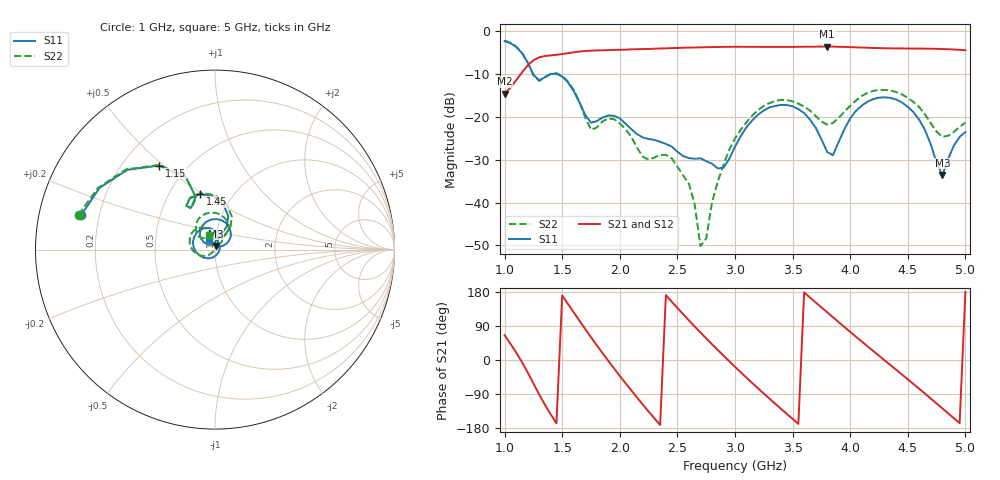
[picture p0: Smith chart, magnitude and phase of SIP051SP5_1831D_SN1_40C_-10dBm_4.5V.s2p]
# GHz  S  dB  R  50
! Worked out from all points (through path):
!   81 points, 1 GHz to 5 GHz, reference 50 ohm
!   highest |S21| = -3.53 dB at 3.8 GHz (marker M1); lowest = -14.5 dB at 1 GHz (marker M2)
!   lowest |S11| = -33.5 dB at 4.8 GHz (marker M3), VSWR 1.04, Z = 50.4 + j2.08 ohm
!   |S11| at or under -10 dB: 1.248 GHz to 1.397 GHz (148.8 MHz wide, 11.2 % of centre); 1.458 GHz to end of sweep
!   |S22| runs from -50.2 to -2.1 dB; largest |S21 - S12| = 0.0027
!   S11 on the Smith chart (normalised r, x): 1 GHz: 0.13, +0.13; 1.15 GHz: 0.35, +0.48; 1.45 GHz: 0.71, +0.49; 5 GHz: 0.93, +0.11
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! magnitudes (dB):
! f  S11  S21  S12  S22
! 1 GHz  -2.3  -14.5  -14.5  -2.1
! 1.15 GHz  -5.0  -9.6  -9.6  -5.0
! 1.3 GHz  -11.4  -6.0  -6.1  -11.6
! 1.45 GHz  -9.9  -5.5  -5.4  -9.7
! 1.7 GHz  -19.5  -4.6  -4.6  -20.1
! 1.75 GHz  -21.3  -4.5  -4.5  -22.9
! 1.95 GHz  -19.7  -4.3  -4.3  -20.5
! 2.2 GHz  -24.8  -4.1  -4.1  -29.3
! 2.35 GHz  -25.8  -4.0  -4.0  -28.9
! 2.6 GHz  -29.6  -3.8  -3.8  -35.6
! 2.7 GHz  -29.6  -3.7  -3.7  -50.2
! 2.75 GHz  -30.3  -3.7  -3.7  -48.4
! 2.9 GHz  -31.8  -3.6  -3.6  -31.2
! 3 GHz  -26.9  -3.6  -3.6  -25.0
! 3.35 GHz  -17.4  -3.6  -3.6  -16.2
! 3.7 GHz  -22.5  -3.5  -3.5  -19.7
! 3.8 GHz  -28.2  -3.5  -3.5  -21.8
! 4.1 GHz  -17.3  -3.8  -3.7  -15.1
! 4.35 GHz  -15.5  -3.9  -4.0  -13.8
! 4.6 GHz  -20.7  -4.0  -4.0  -17.7
! 4.8 GHz  -33.5  -4.1  -4.1  -24.6
! 5 GHz  -23.5  -4.4  -4.4  -21.3
